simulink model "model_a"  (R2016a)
settings: Solver=FixedStepAuto  StartTime=0.0  StopTime=0.1  RelTol=1e-3
PreLoadFcn:
  | % ---  DO NOT REMOVE THIS CODE (2025.1)   ---
  |     % create Simulink variants
  |     if not(exist('variant_simulation', 'var'))
  |         variant_simulation = Simulink.Variant('SIMULINK_MODE==0');
  |     end
  |     if not(exist('variant_generation', 'var'))
  |         variant_generation = Simulink.Variant('SIMULINK_MODE==1');
  |     end
  | 
  |     % check SDK version
  |     required_lib_version = 3900.3;
  |     required_lib_ver_str = '2025.1';
  |     lib_path = [getenv('IX_SIMULINK_ACG_BB_3') '\simulink\blocks\BoomBox.slx'];
  |     if exist(lib_path, 'file')
  |         lib_version = str2double(Simulink.MDLInfo(lib_path).ModelVersion); % fullpath to avoid getting shadowing files
  |         if lib_version < required_lib_version || isnan(lib_version)
  |             error(['The model ''' bdroot ''' has been saved with a more recent version of ACG SDK (' required_lib_ver_str ') and might not work as expected. <a href="matlab:private_end_string = ''--- PLACE YOUR CODE BELOW THIS LINE ---'';private_fcn = get_param(bdroot, ''PreLoadFcn'');private_end_index = strfind(private_fcn, private_end_string);set_param(bdroot, ''PreLoadFcn'', strtrim(private_fcn(private_end_index(end)+length(private_end_string):end)));private_fcn = get_param(bdroot, ''PostLoadFcn'');private_end_index = strfind(private_fcn, private_end_string);set_param(bdroot, ''PostLoadFcn'', strtrim(private_fcn(private_end_index(end)+length(private_end_string):end)));private_fcn = get_param(bdroot, ''InitFcn'');private_end_index = strfind(private_fcn, private_end_string);set_param(bdroot, ''InitFcn'', strtrim(private_fcn(private_end_index(end)+length(private_end_string):end)));clear private_end_string private_fcn private_end_index;open(bdroot);">Click here</a> to continue anyway, or download the latest version of the SDK at <a href="www.imperix.com/downloads">www.imperix.ch/downloads</a>.']);
  |         end
  |     elseif exist(getenv('IX_SIMULINK_ACG_BB_3'), 'dir')
  |         error(['Library file for imperix ACG SDK not found in path ''' lib_path '''. Please try to re-install ACG SDK (<a href="www.imperix.com/downloads">www.imperix.ch/downloads</a>).']);
  |     else
  |         error('ACG SDK is not installed on this computer and the model will not work as expected. Please download ACG SDK at <a href="www.imperix.com/downloads">www.imperix.ch/downloads</a>, install it, and reopen the model.');
  |     end
  |     clear required_lib_version required_lib_ver_str lib_path lib_version;
  | 
  |     ix_acg_path = getenv('IX_SIMULINK_ACG_BB_3');
  |     addpath(fullfile(ix_acg_path, 'simulink\target'));
  |     addpath(fullfile(ix_acg_path, 'simulink\blocks'));
  |     addpath(fullfile(ix_acg_path, 'simulink\functions'));
  |     sl_refresh_customizations;
  |     clear ix_acg_path;
  | 
  |     % The SIMULINK_MODE variable is created in the base
  |     % workspace in the PostLoadFcn from the block whose id is kb0101
  |     % All opened models share a common variant configuration.
  | 
  |     Model_PreLoadFcn(bdroot);
  | % --- PLACE YOUR CODE BELOW THIS LINE ---
PostLoadFcn:
  | % ---  DO NOT REMOVE THIS CODE (2025.1)   ---
  |     % change the execution mode of simulink depending on the radio button:
  |     if(strcmp('Automated Code Generation',get_param(Find_imperix_blocks(bdroot,'Configuration'),'SLMODE')))
  |         assignin('base', 'SIMULINK_MODE', 1);
  |     else
  |         assignin('base', 'SIMULINK_MODE', 0);
  |     end
  | 
  |     Model_PostLoadFcn(bdroot);
  | % --- PLACE YOUR CODE BELOW THIS LINE ---
InitFcn:
  | % ---  DO NOT REMOVE THIS CODE (2025.1)   ---
  |     % check SDK version
  |     required_lib_version = 3900.3;
  |     required_lib_ver_str = '2025.1';
  |     lib_path = [getenv('IX_SIMULINK_ACG_BB_3') '\simulink\blocks\BoomBox.slx'];
  |     if exist(lib_path, 'file')
  |         lib_version = str2double(Simulink.MDLInfo(lib_path).ModelVersion); % fullpath to avoid getting shadowing files
  |         if lib_version < required_lib_version || isnan(lib_version)
  |             error(['The model ''' bdroot ''' has been saved with a more recent version of ACG SDK (' required_lib_ver_str ') and might not work as expected. <a href="matlab:private_end_string = ''--- PLACE YOUR CODE BELOW THIS LINE ---'';private_fcn = get_param(bdroot, ''PreLoadFcn'');private_end_index = strfind(private_fcn, private_end_string);set_param(bdroot, ''PreLoadFcn'', strtrim(private_fcn(private_end_index(end)+length(private_end_string):end)));private_fcn = get_param(bdroot, ''PostLoadFcn'');private_end_index = strfind(private_fcn, private_end_string);set_param(bdroot, ''PostLoadFcn'', strtrim(private_fcn(private_end_index(end)+length(private_end_string):end)));private_fcn = get_param(bdroot, ''InitFcn'');private_end_index = strfind(private_fcn, private_end_string);set_param(bdroot, ''InitFcn'', strtrim(private_fcn(private_end_index(end)+length(private_end_string):end)));clear private_end_string private_fcn private_end_index;open(bdroot);">Click here</a> to continue anyway, or download the latest version of the SDK at <a href="www.imperix.com/downloads">www.imperix.ch/downloads</a>.']);
  |         end
  |     elseif exist(getenv('IX_SIMULINK_ACG_BB_3'), 'dir')
  |         error(['Library file for imperix ACG SDK not found in path ''' lib_path '''. Please try to re-install ACG SDK (<a href="www.imperix.com/downloads">www.imperix.ch/downloads</a>).']);
  |     else
  |         error('ACG SDK is not installed on this computer and the model will not work as expected. Please download ACG SDK at <a href="www.imperix.com/downloads">www.imperix.ch/downloads</a>, install it, and reopen the model.');
  |     end
  |     clear required_lib_version required_lib_ver_str lib_path lib_version;
  | 
  |     Model_InitFcn(bdroot);
  | % --- PLACE YOUR CODE BELOW THIS LINE ---
model workspace (MAT data in the model file):
  CTRLPERIOD = 5e-05
  MODEL_ARG = 0
  TSAMPLE = 2e-06
  global_CLK_number = 0
  global_INT_number = 1
  global_SVM_instance_id = 0
  global_can_baud_rate = '1000000'
  global_comp_time = 0.2
  global_cycle_delay = 1e-05
  global_ip_addresses : cell (value not decoded)
  imperix_block_list : cell (value not decoded)
undefined symbols (not defined in the file): B, Board, Box, byte, Micro, ns, PRO, RCP, TPI
libraries: BoomBox x3

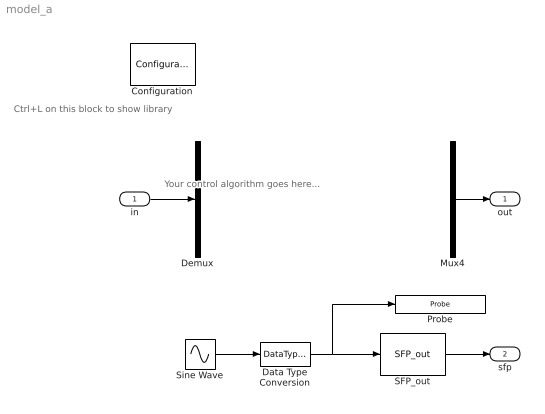
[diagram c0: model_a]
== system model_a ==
  note: Your control algorithm goes here...
  note: Ctrl+L on this block to show library
  in : Inport
  Configuration : BoomBox/Configuration  Description=Please leave the Priority (below parameter) to maximum negative to ensure that this block is always executed first.  Priority=-99999  SLMODE=Automated Code Generation  load_from_file=off  init_file=param.m  clk0_freq=20e3  interrupt_phase=0.5  interrupt_pstsclr=0  clk0_is_variable=off  sampling_conf=Disabled  nb_oversamples=0  sampling_phases=[0.2 0.8]  adc_delay_conf=2000 ns (B-Box RCP, B-Box Micro, B-Board PRO or TPI)  custom_adc_delay=off  adc_delay_s=500e-9  Parameter15=0  MAXSTEP=auto  MINSTEP=auto  RELTOL=1e-3  TSAMPLE=2e-6  computation_time=0.2  cycle_delay_unit=Period  powerlib_model=(A) Simple  powerlib_switch=Switching devices (switched)  powerlib_pwm=PWM signals  KBID=kb0101  interrupt_presc_real=1  interrupt_ticks_real=12500  highest_device_id=0
  Data Type Conversion : DataTypeConversion  OutDataTypeStr=single
  Demux : Demux  Outputs=5
  Mux4 : Mux  Inputs=5
  Probe : BoomBox/Probe  VARNAME=sine_wave_out  EVALUATE=Literal  DATATYPE=single  CAN_ENABLED=off  CAN_ADDRESS=0  CAN_TX_FREQ=10  init_baudrate=0  CAN_BAUDRATE=1000000  can_endianness=Little-endian  ETH_ENABLED=off  ETH_PORT=2000  ETH_IP_LIST=IP address 0  eth_endianness=Little-endian  ETH_TX_FREQ=10  init_ip=0  KBID=kb0502  CAN_BIG_ENDIAN=0  ETH_BIG_ENDIAN=0  ETH_IP_SFCN=empty  CAN_MB_ID=0  ETH_MB_ID=1  RESIZE=0
  SFP_out : BoomBox/SFP_out  CHANNEL_NAME=name  EVALUATE=Literal  NBR_SIGNALS=1  SIGNAL_TYPE=int8 (1 byte)  TRANS_MODE=None (send all data)  SIM_OUT=on  MB_ID=0  OPERATING_MODE=0  KBID=kb0305
  Sine Wave : Sin  Frequency=2*pi*50  SampleTime=CTRLPERIOD
  out : Outport
  sfp : Outport  Port=2
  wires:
  in/1 -> Demux/1
  Mux4/1 -> out/1
  Configuration/2 -> ?  "to ADC blocks"
  Configuration/1 -> ?  "to PWM blocks"
  Sine Wave/1 -> Data Type Conversion/1
  SFP_out/1 -> sfp/1
  Data Type Conversion/1 -> Probe/1, SFP_out/1
